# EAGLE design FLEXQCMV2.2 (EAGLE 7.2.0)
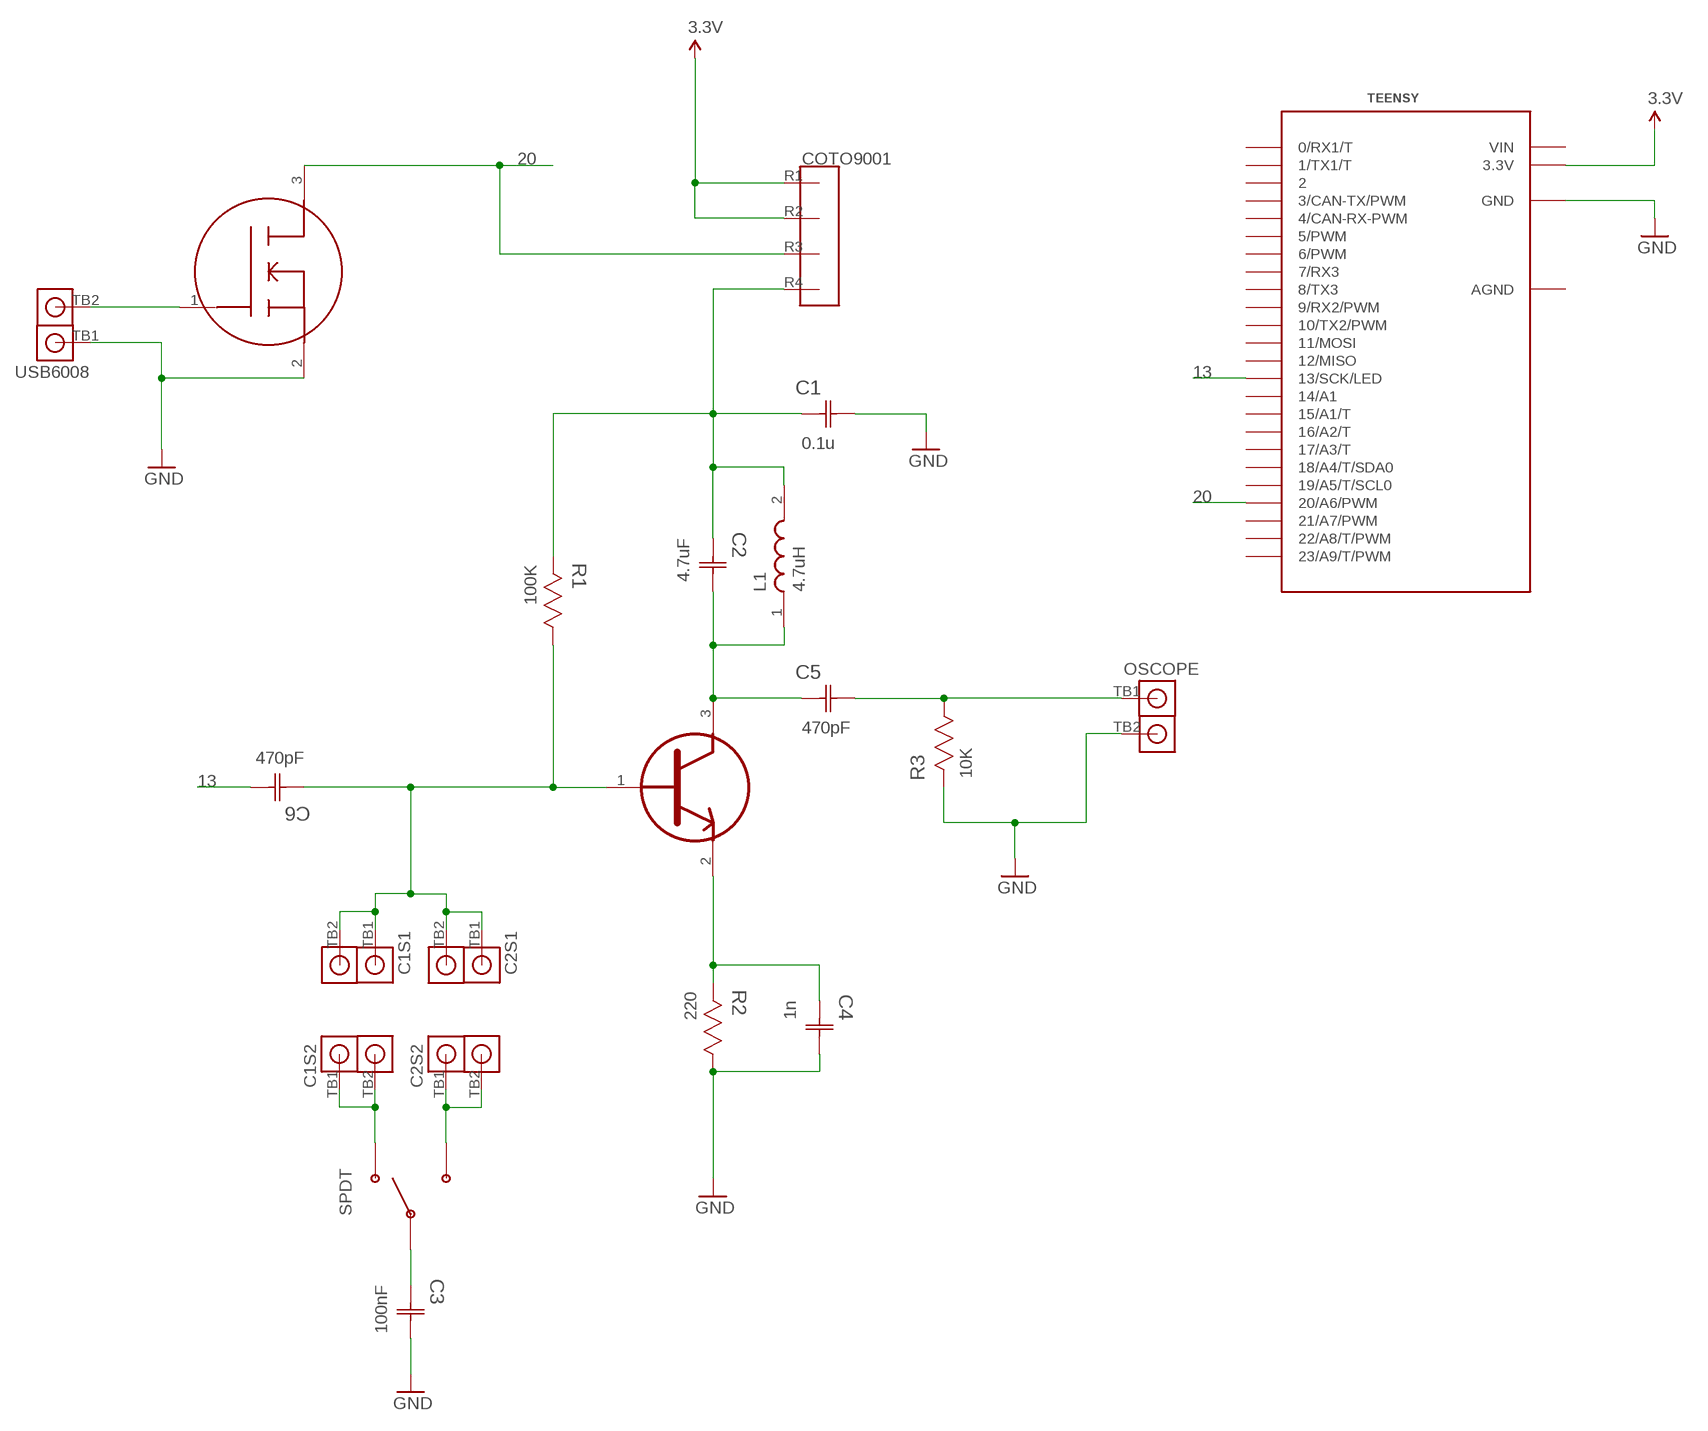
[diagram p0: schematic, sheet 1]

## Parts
C1  0.1u  C1206C104K1RACTU  [CAPC3216X88N]
C1S1  TERMBLOCKX2  [TERMBLOCKX2]
C1S2  TERMBLOCKX2  [TERMBLOCKX2]
C2  4.7uF  C1206C475K3RACTU  [CAPC3216X180N]
C2S1  TERMBLOCKX2  [TERMBLOCKX2]
C2S2  TERMBLOCKX2  [TERMBLOCKX2]
C3  100nF  C1206C104K1RACTU  [CAPC3216X88N]
C4  1n  C1206C103K5RACTU  [CAPC3216X88N]
C5  470pF  C1206C474K3RACTU  [CAPC3216X100N]
C6  470pF  C1206C474K3RACTU  [CAPC3216X100N]
COTO9001  COTO9001  [COTO9001]
L1  4.7uH  B82422A1472K100  [INDC3225X210N]
OSCOPE  TERMBLOCKX2  [TERMBLOCKX2]
R1  100K  CRCW1206100KJNEA  [RESC3216X71N]
R2  220  CRCW1206220RJNEA  [RESC3216X71N]
R3  10K  CRCW120610K0FKEA  [RESC3216X71N]
SPDT  SPDTSWITCH  [SPDTSWITCH]
TEENSY  TEENSY_3.1_DIL  [TEENSY3-DIL]
U1  FET  2N7002K  [SOT95P230X110-3N]
U2  BJT  BC847C  [SOT95P230X110-3N]
USB6008  TERMBLOCKX2  [TERMBLOCKX2]

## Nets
3.3V: COTO9001.R1 COTO9001.R2 TEENSY.3.3V
13: C6.2(C2) TEENSY.13(13/SCK/LED)
20: COTO9001.R3 TEENSY.20/A6(20/A6/PWM) U1.3(D)
GND: C1.2(C2) C3.2(C2) C4.2(C2) OSCOPE.TB2 R2.1 R3.2 TEENSY.GND U1.2(S) USB6008.TB1
N$1: U1.1(G) USB6008.TB2
N$2: C4.1(C1) R2.2 U2.2(E)
N$3: C1S2.TB1 C1S2.TB2 SPDT.SW1
N$4: C1.1(C1) C2.1(C1) COTO9001.R4 L1.2 R1.2
N$5: C1S1.TB1 C1S1.TB2 C2S1.TB1 C2S1.TB2 C6.1(C1) R1.1 U2.1(B)
N$6: C3.1(C1) SPDT.SW2
N$7: C2S2.TB1 C2S2.TB2 SPDT.SW3
N$9: C2.2(C2) C5.1(C1) L1.1 U2.3(C)
N$11: C5.2(C2) OSCOPE.TB1 R3.1
Unconnected: TEENSY.0(0/RX1/T) TEENSY.1(1/TX1/T) TEENSY.2 TEENSY.3(3/CAN-TX/PWM) TEENSY.4(4/CAN-RX-PWM) TEENSY.5(5/PWM) TEENSY.6(6/PWM) TEENSY.7(7/RX3) TEENSY.8(8/TX3) TEENSY.9(9/RX2/PWM) TEENSY.10(10/TX2/PWM) TEENSY.11(11/MOSI) TEENSY.12(12/MISO) TEENSY.14/A0(14/A1) TEENSY.15/A1(15/A1/T) TEENSY.16/A2(16/A2/T) TEENSY.17/A3(17/A3/T) TEENSY.18/A4(18/A4/T/SDA0) TEENSY.19/A5(19/A5/T/SCL0) TEENSY.21/A7(21/A7/PWM) TEENSY.22/A8(22/A8/T/PWM) TEENSY.23/A9(23/A9/T/PWM)

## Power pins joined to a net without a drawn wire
AGND: TEENSY.AGND
VIN: TEENSY.VIN

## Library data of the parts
C1 = Kemet_By_element14_Batch_1:C1206C104K1RACTU: CAPACITOR, 1206; MPN: C1206C104K1RACTU; OC_FARNELL: 1414714; OC_NEWARK: 85C2205; SUPPLIER: Kemet; TOLERANCE: ±10%; VALUE: 100nF; VOLTAGERATING: 100V
C1S1 C1S2 C2S1 C2S2 OSCOPE USB6008 = FLEXQCMLIBRARY:TERMBLOCKX2
C2 = Kemet_By_element14_Batch_1:C1206C475K3RACTU: CAPACITOR, 1206; MPN: C1206C475K3RACTU; OC_FARNELL: 1288211; OC_NEWARK: 88K0224; SUPPLIER: Kemet; TOLERANCE: ±10%; VOLTAGERATING: 25V
C3 = Kemet_By_element14_Batch_1:C1206C104K1RACTU: CAPACITOR, 1206; MPN: C1206C104K1RACTU; OC_FARNELL: 1414714; OC_NEWARK: 85C2205; SUPPLIER: Kemet; TOLERANCE: ±10%; VOLTAGERATING: 100V
C4 = Kemet_By_element14_Batch_1:C1206C103K5RACTU: CAPACITOR, 1206; MPN: C1206C103K5RACTU; OC_FARNELL: 1414713; OC_NEWARK: 61H7741; SUPPLIER: Kemet; TOLERANCE: ±10%; VALUE: 10nF; VOLTAGERATING: 50V
C5 C6 = Kemet_By_element14_Batch_1:C1206C474K3RACTU: CAPACITOR, 1206; MPN: C1206C474K3RACTU; OC_FARNELL: 1288280; OC_NEWARK: 25M8811; SUPPLIER: Kemet; TOLERANCE: ±10%; VALUE: 470nF; VOLTAGERATING: 25V
COTO9001 = FLEXQCMLIBRARY:COTO9001
L1 = Epcos_By_element14_Batch_1:B82422A1472K100: SMT inductors; MPN: B82422A1472K100; OC_FARNELL: 1644345; OC_NEWARK: 22C0379; SUPPLIER: EPCOS; TOLERANCE: ±10%
R1 = Vishay_By_element14_Batch_1:CRCW1206100KJNEA: RESISTOR, 1206; MPN: CRCW1206100KJNEA; OC_FARNELL: 1534576; OC_NEWARK: 59M6947; SUPPLIER: Vishay; TOLERANCE: ±5%; VALUE: 100K Ohms; WATTAGE: 0.25W
R2 = Vishay_By_element14_Batch_1:CRCW1206220RJNEA: RESISTOR, 1206; MPN: CRCW1206220RJNEA; OC_FARNELL: -; OC_NEWARK: 59M6970; SUPPLIER: Vishay; TOLERANCE: ±5%; VALUE: 220 Ohms; WATTAGE: 0.25W
R3 = Vishay_By_element14_Batch_1:CRCW120610K0FKEA: RESISTOR, 1206; MPN: CRCW120610K0FKEA; OC_FARNELL: 1469970; OC_NEWARK: 53K1907; SUPPLIER: Vishay; TOLERANCE: ±1%; VALUE: 10K Ohms; WATTAGE: 0.25W
SPDT = FLEXQCMLIBRARY:SPDTSWITCH
TEENSY = Teensy_3_and_LC_Series_Boards_v1.0:TEENSY_3.1_DIL: Teensy 3.1 or 3.2 in a DIL Layout.
U1 = NXP_By_element14_Batch_1:2N7002K: logic level FET; MPN: 2N7002K; OC_FARNELL: 1758065; OC_NEWARK: -; PACKAGE: SOT-3; SUPPLIER: NXP Semiconductors
U2 = NXP_By_element14_Batch_1:BC847C

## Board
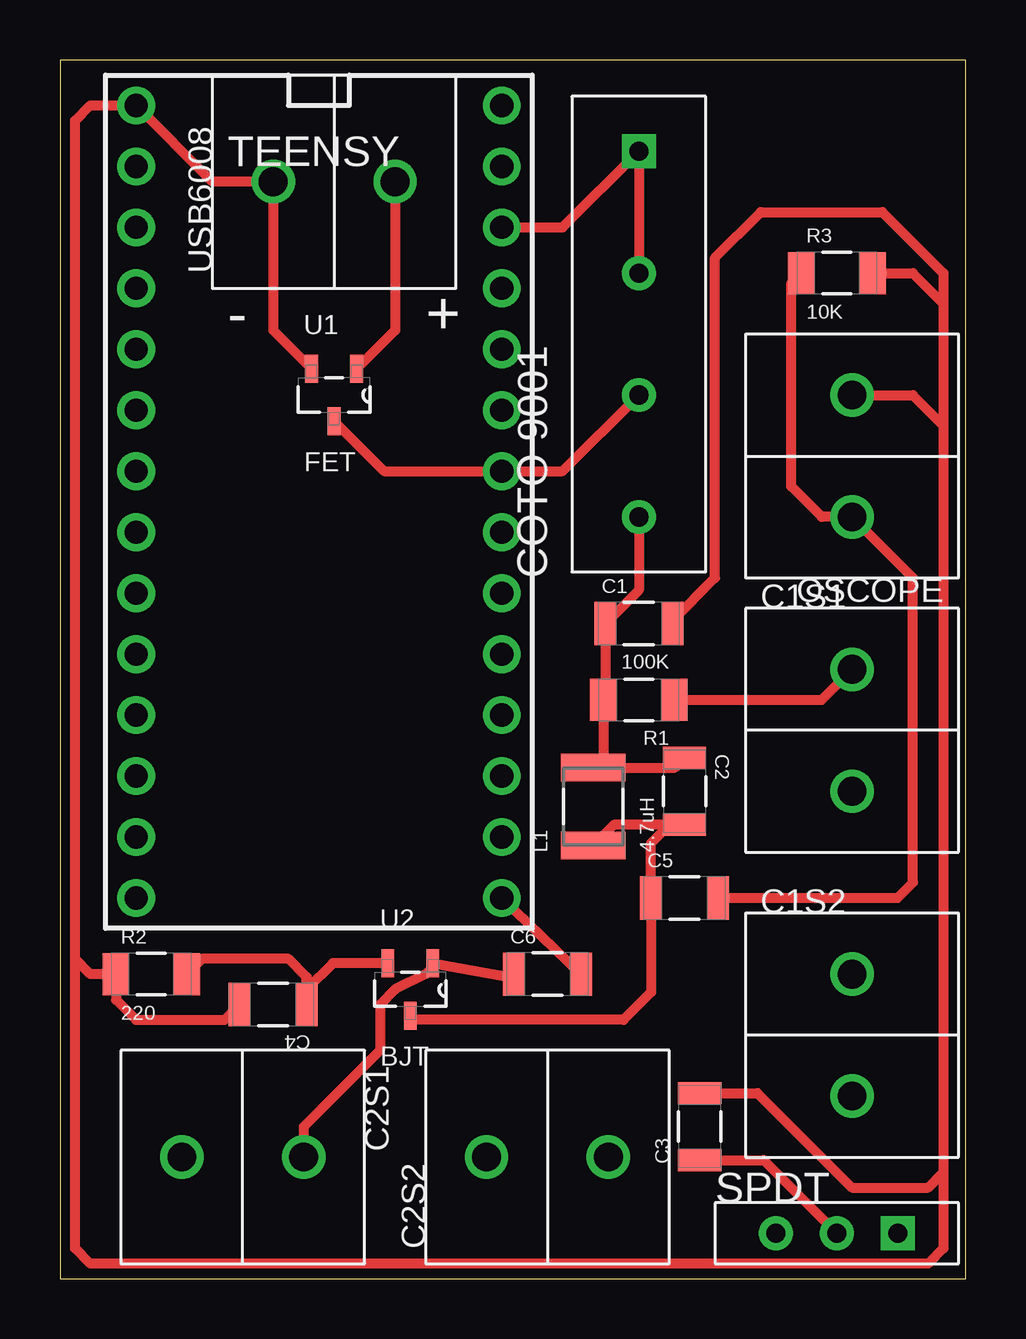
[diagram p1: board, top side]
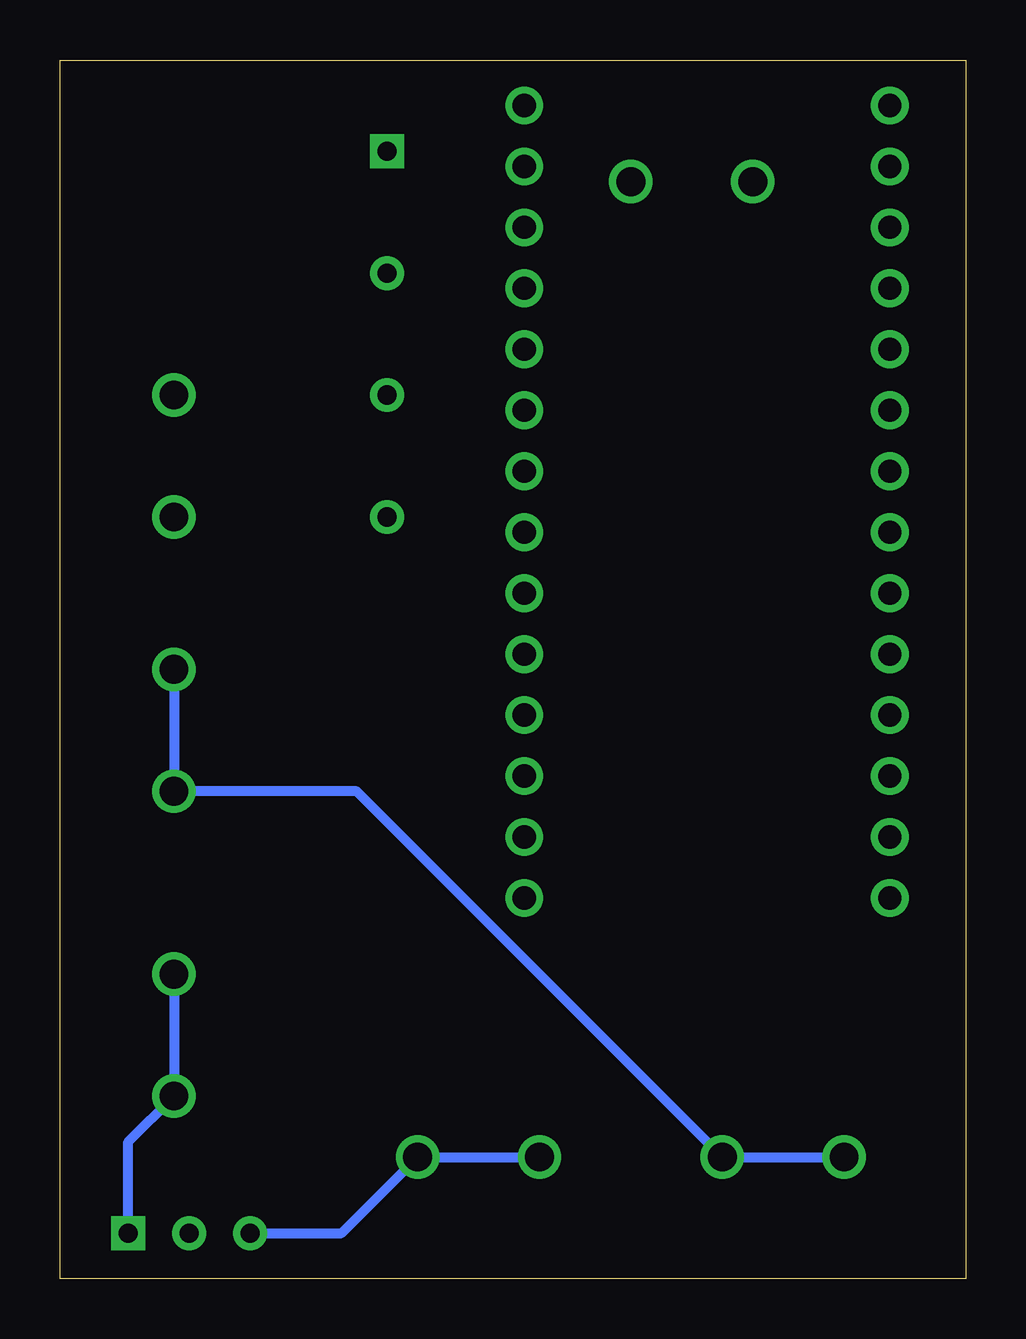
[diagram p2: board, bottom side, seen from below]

Size 37.77 x 50.79 mm. Coordinates in mm from the lower left corner, seen from the top.
Outline: 0,0 37.77,0 37.77,50.79 0,50.79 0,0
Copper layers (1*16): Top 0.035mm / dielectric 1.5mm / Bottom 0.035mm
Design rules "SparkFun": minimum track width 8mil, minimum drill 20mil, track to track 8mil, track to pad 8mil, pad to pad 8mil, via to via 8mil, smd to smd 8mil, copper to edge 10mil, drill to drill 8mil, minimum pad ring 12mil, minimum via ring 10mil, stop-mask expansion 4mil, vias tented up to drill 25mil, thermal gap 10mil

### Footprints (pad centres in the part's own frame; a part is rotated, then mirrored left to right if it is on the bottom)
CAPC3216X88N = smd 0.914 x 1.803: 1 -1.397,0; 2 1.397,0
TERMBLOCKX2 = drill 1.2: TB1 0,2.54; TB2 0,-2.54
CAPC3216X180N = smd 0.914 x 1.803: 1 -1.397,0; 2 1.397,0
CAPC3216X100N = smd 0.914 x 1.803: 1 -1.397,0; 2 1.397,0
COTO9001 = drill 0.8 square: R1 0,7.62 | drill 0.8: R2 0,2.54; R3 0,-2.54; R4 0,-7.62
INDC3225X210N = smd 1.143 x 2.692: 1 -1.626,0; 2 1.626,0
RESC3216X71N = smd 1.118 x 1.753: 1 -1.473,0; 2 1.473,0
SPDTSWITCH = drill 0.8 square: SW1 0,2.54 | drill 0.8: SW2 0,0; SW3 0,-2.54
TEENSY3-DIL = drill 0.965: 0 -7.62,13.97; 1 -7.62,11.43; 2 -7.62,8.89; 3 -7.62,6.35; 3.3V 7.62,11.43; 4 -7.62,3.81; 5 -7.62,1.27; 6 -7.62,-1.27; 7 -7.62,-3.81; 8 -7.62,-6.35; 9 -7.62,-8.89; 10 -7.62,-11.43; 11 -7.62,-13.97; 12 -7.62,-16.51; 13 7.62,-16.51; 14/A0 7.62,-13.97; 15/A1 7.62,-11.43; 16/A2 7.62,-8.89; 17/A3 7.62,-6.35; 18/A4 7.62,-3.81; 19/A5 7.62,-1.27; 20/A6 7.62,1.27; 21/A7 7.62,3.81; 22/A8 7.62,6.35; 23/A9 7.62,8.89; AGND 7.62,13.97; GND -7.62,16.51; VIN 7.62,16.51
SOT95P230X110-3N = smd 1.168 x 0.533: 1 -1.092,0.94; 2 -1.092,-0.94; 3 1.092,0

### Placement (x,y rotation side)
C1  24.13,27.3 0 top
C1S1  33.02,22.86 0 top
C1S2  33.02,10.16 0 top
C2  26.04,20.32 270 top
C2S1  7.62,5.08 270 top
C2S2  20.32,5.08 90 top
C3  26.67,6.35 90 top
C4  8.89,11.43 180 top
C5  26.04,15.88 0 top
C6  20.32,12.7 0 top
COTO9001  24.13,39.37 0 top
L1  22.23,19.68 90 top
OSCOPE  33.02,34.29 180 top
R1  24.13,24.13 180 top
R2  3.81,12.7 0 top
R3  32.38,41.91 0 top
SPDT  32.38,1.91 270 top
TEENSY  10.79,32.38 0 top
U1  11.43,36.83 270 top
U2  14.61,12.06 270 top
USB6008  11.43,45.72 90 top

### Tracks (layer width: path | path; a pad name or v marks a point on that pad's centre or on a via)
3.3V
  Top 0.406: TEENSY.3.3V 20.95,43.81 COTO9001.R1 COTO9001.R2
13
  Top 0.406: TEENSY.13 C6.2
20
  Top 0.406: U1.3 13.51,33.66 TEENSY.20/A6 20.95,33.66 COTO9001.R3
GND
  Top 0.406: U1.2 8.89,39.52 USB6008.TB1 6.35,45.72 TEENSY.GND 1.27,48.9 0.64,48.26 0.64,13.34 | OSCOPE.TB2 35.56,36.83 36.83,35.56 | 36.83,35.56 36.83,4.45 | 36.83,4.45 36.83,1.27 36.2,0.64 1.27,0.64 0.64,1.27 0.64,13.34 | R3.2 35.56,41.91 36.83,40.64 | 36.83,40.64 36.83,35.56 | 0.64,13.34 1.27,12.7 R2.1 2.34,11.63 3.17,10.79 6.86,10.79 C4.2 | C3.2 29.08,7.75 33.02,3.81 36.2,3.81 36.83,4.45 | C1.2 25.53,27.43 27.3,29.21 27.3,42.55 29.21,44.45 34.29,44.45 36.83,41.91 36.83,40.64
N$1
  Top 0.406: USB6008.TB2 13.97,39.52 U1.1
N$2
  Top 0.406: C4.1 10.29,12.06 | 10.29,12.06 10.29,12.57 9.53,13.34 5.92,13.34 R2.2 | U2.2 11.38,13.16 10.29,12.06
N$3
  Bottom 0.406: C1S2.TB1 C1S2.TB2 34.92,5.71 SPDT.SW1
N$4
  Top 0.406: COTO9001.R4 24.13,28.7 C1.1 22.73,24.21 R1.2 22.66,21.74 L1.2 25.63,21.31 C2.1
N$5
  Top 0.406: C6.1 18.8,12.57 U2.1 15.54,13.01 15.24,12.7 13.97,12.06 13.34,11.43 13.34,9.53 10.16,6.35 C2S1.TB1 | R1.1 31.75,24.13 C1S1.TB1
  Bottom 0.406: C1S1.TB1 C1S1.TB2 25.4,20.32 C2S1.TB1 C2S1.TB2
N$6
  Top 0.406: C3.1 29.34,4.95 SPDT.SW2
N$7
  Bottom 0.406: SPDT.SW3 26.04,1.91 C2S2.TB2 C2S2.TB1
N$9
  Top 0.406: C2.2 25.4,18.92 | 25.4,18.92 23.09,18.92 L1.1 | U2.3 14.78,10.79 23.5,10.79 24.64,11.94 C5.1 24.64,18.16 25.4,18.92
N$11
  Top 0.406: C5.2 34.92,15.88 35.56,16.51 35.56,29.21 OSCOPE.TB1 31.75,31.75 30.48,33.02 30.48,41.48 R3.1

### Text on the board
tPlace: - | +

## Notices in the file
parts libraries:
SparkFun-Aesthetics: Licensing: Creative Commons ShareAlike 4.0 International - https://creativecommons.org/licenses/by-sa/4.0
